(* Logix 5000 AddOnInstructionDefinition export B256_EtoC; software revision 30.00 *)

ADD_ON_INSTRUCTION D_SHR   (* revision 1.0, vendor Ken Fischer, NSWCPD, C512 *)
// DINT bit shift right of the 32-bit argument Inp_A by Inp_B bits with paddding by zeros on the right
// Revision note:
// Rev1.0: TBD - Initial Release
VAR_IN_OUT
   Inp_A : DINT; {required}   // 64-bit Integer to be right circular rotated
END_VAR
VAR_INPUT
   Inp_B : INT; {required}   // Number of bits to shift
END_VAR
VAR_IN_OUT
   Out : DINT; {required}   // Result
END_VAR
VAR
   BSR_Cntrl : CONTROL := (LEN := 32);
   ONS : BOOL;
   Source_Bit : BOOL;
   Wrk_InpA : DINT[2];
END_VAR

ROUTINE Logic   (* ladder *)
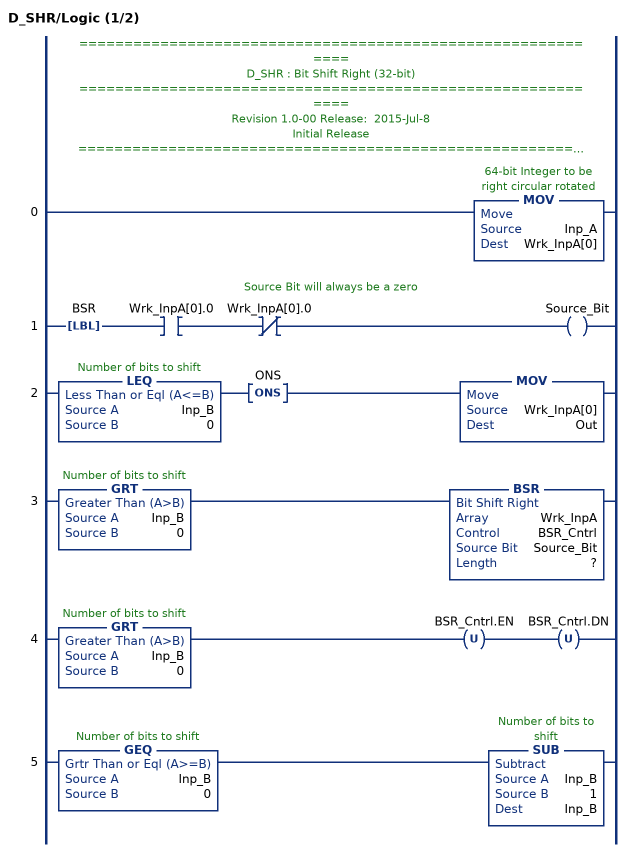
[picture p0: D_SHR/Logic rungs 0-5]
   // ============================================================
   // D_SHR : Bit Shift Right (32-bit)
   // ============================================================
   // Revision 1.0-00 Release:  2015-Jul-8
   // Initial Release
   // ============================================================
   // Performs a right bit shift of the 32-bit argument Inp_A by the
   // number of bits defined in the 16-bit argument Inp_B, with padding by zeros.
   0: MOV(Inp_A,Wrk_InpA[0]);
   // Source Bit will always be a zero
   1: LBL(BSR)XIC(Wrk_InpA[0].0)XIO(Wrk_InpA[0].0)OTE(Source_Bit);
   2: LEQ(Inp_B,0)ONS(ONS)MOV(Wrk_InpA[0],Out);
   3: GRT(Inp_B,0)BSR(Wrk_InpA,BSR_Cntrl,Source_Bit,?);
   4: GRT(Inp_B,0)OTU(BSR_Cntrl.EN)OTU(BSR_Cntrl.DN);
   5: GEQ(Inp_B,0)SUB(Inp_B,1,Inp_B);
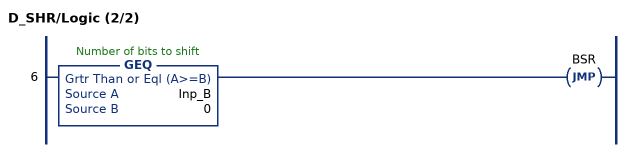
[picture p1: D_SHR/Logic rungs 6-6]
   6: GEQ(Inp_B,0)JMP(BSR);
END_ROUTINE
END_ADD_ON_INSTRUCTION

ADD_ON_INSTRUCTION D_SHL   (* revision 1.0, vendor Ken Fischer, NSWCPD, C512 *)
// DINT bit shift left of the 32-bit argument Inp_A by Inp_B bits with paddding by zeros on the right
// Revision note:
// Rev1.0: TBD - Initial Release
VAR_IN_OUT
   Inp_A : DINT; {required}   // 64-bit Integer to be right circular rotated
END_VAR
VAR_INPUT
   Inp_B : INT; {required}   // Number of bits to shift
END_VAR
VAR_IN_OUT
   Out : DINT; {required}   // Result
END_VAR
VAR
   Wrk_InpA : DINT[2];
   Source_Bit : BOOL;
   ONS : BOOL;
   BSL_Cntrl : CONTROL := (LEN := 32);
END_VAR

ROUTINE Logic   (* ladder *)
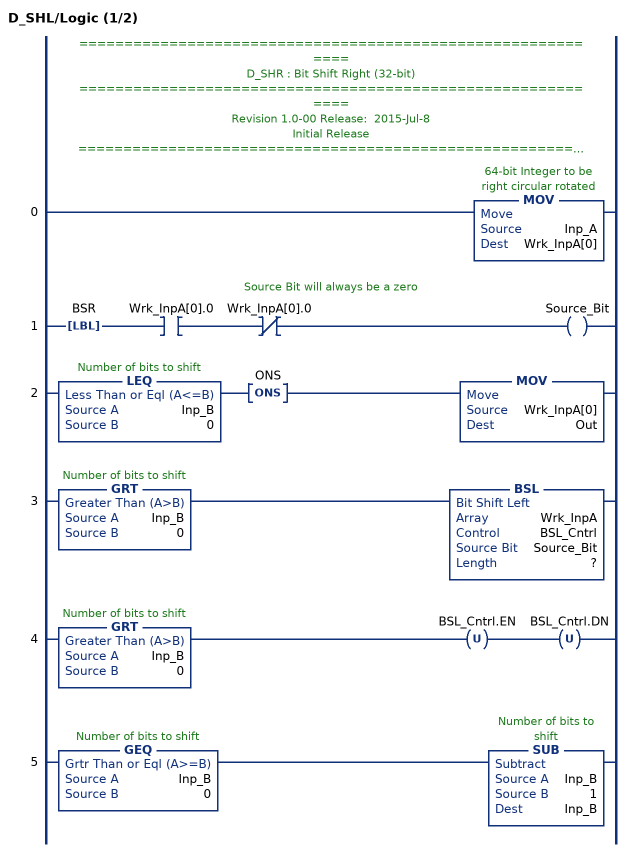
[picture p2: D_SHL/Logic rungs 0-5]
   // ============================================================
   // D_SHR : Bit Shift Right (32-bit)
   // ============================================================
   // Revision 1.0-00 Release:  2015-Jul-8
   // Initial Release
   // ============================================================
   // Performs a left bit shift of the 32-bit argument Inp_A by the
   // number of bits defined in the 16-bit argument Inp_B, with padding by zeros.
   0: MOV(Inp_A,Wrk_InpA[0]);
   // Source Bit will always be a zero
   1: LBL(BSR)XIC(Wrk_InpA[0].0)XIO(Wrk_InpA[0].0)OTE(Source_Bit);
   2: LEQ(Inp_B,0)ONS(ONS)MOV(Wrk_InpA[0],Out);
   3: GRT(Inp_B,0)BSL(Wrk_InpA,BSL_Cntrl,Source_Bit,?);
   4: GRT(Inp_B,0)OTU(BSL_Cntrl.EN)OTU(BSL_Cntrl.DN);
   5: GEQ(Inp_B,0)SUB(Inp_B,1,Inp_B);
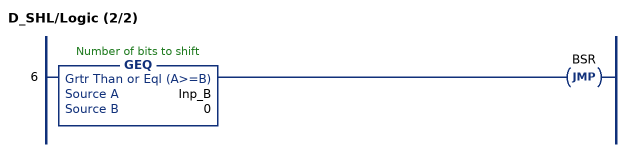
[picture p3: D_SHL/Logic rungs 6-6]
   6: GEQ(Inp_B,0)JMP(BSR);
END_ROUTINE
END_ADD_ON_INSTRUCTION

ADD_ON_INSTRUCTION B256_EtoC   (* revision 1.0 20170916, vendor Kenneth A. Fischer *)
// Convert 256-bit value using 32 8-bit pieces into 256-bit value using 22 12-bit pieces
// Revision note:
// Rev1.0: 20170916 - Initial Release
VAR_IN_OUT
   Inp_E : DINT[32]; {required}
   Out_C : DINT[22]; {required}
END_VAR
VAR
   i : INT;
   j : INT;
   TEMP1 : DINT;
   TEMP2 : DINT;
   D_SHL : D_SHL;
   D_SHR : D_SHR;
END_VAR

ROUTINE Logic   (* ladder *)
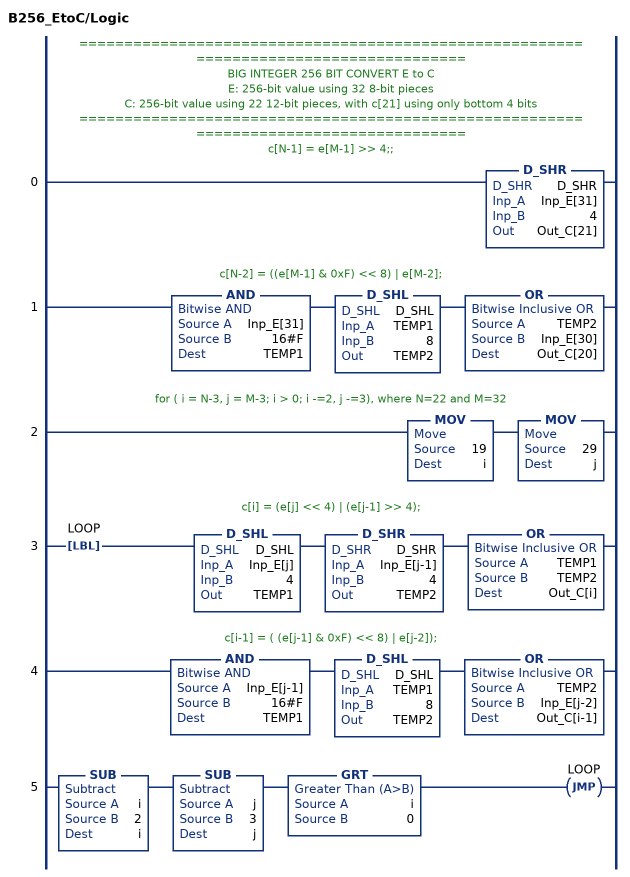
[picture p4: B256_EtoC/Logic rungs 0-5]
   // ======================================================================================
   // BIG INTEGER 256 BIT CONVERT E to C
   // E: 256-bit value using 32 8-bit pieces
   // C: 256-bit value using 22 12-bit pieces, with c[21] using only bottom 4 bits
   // ======================================================================================
   // c[N-1] = e[M-1] >> 4;;
   0: D_SHR(D_SHR,Inp_E[31],4,Out_C[21]);
   // c[N-2] = ((e[M-1] & 0xF) << 8) | e[M-2];
   1: AND(Inp_E[31],16#F,TEMP1)D_SHL(D_SHL,TEMP1,8,TEMP2)OR(TEMP2,Inp_E[30],Out_C[20]);
   // for ( i = N-3, j = M-3; i > 0; i -=2, j -=3), where N=22 and M=32
   2: MOV(19,i)MOV(29,j);
   // c[i] = (e[j] << 4) | (e[j-1] >> 4);
   3: LBL(LOOP)D_SHL(D_SHL,Inp_E[j],4,TEMP1)D_SHR(D_SHR,Inp_E[j-1],4,TEMP2)OR(TEMP1,TEMP2,Out_C[i]);
   // c[i-1] = ( (e[j-1] & 0xF) << 8) | e[j-2]);
   4: AND(Inp_E[j-1],16#F,TEMP1)D_SHL(D_SHL,TEMP1,8,TEMP2)OR(TEMP2,Inp_E[j-2],Out_C[i-1]);
   5: SUB(i,2,i)SUB(j,3,j)GRT(i,0)JMP(LOOP);
END_ROUTINE
END_ADD_ON_INSTRUCTION
